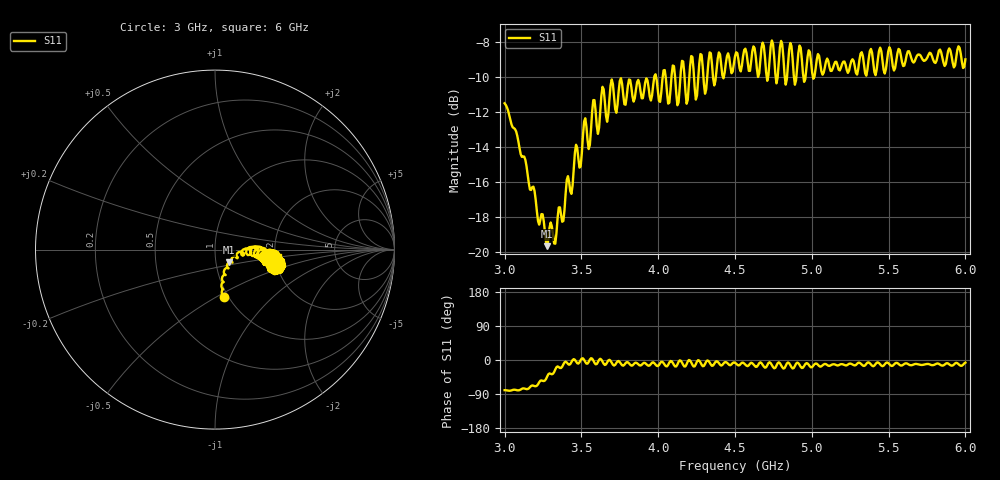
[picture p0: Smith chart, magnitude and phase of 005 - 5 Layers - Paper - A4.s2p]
!  02/07/2025  15:59:35
! Ref Plane: 0.000 mm
# MHZ S MA R  50
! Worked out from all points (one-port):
!   401 points, 3 GHz to 6 GHz, reference 50 ohm
!   lowest |S11| = -19.7 dB at 3.277 GHz (marker M1), VSWR 1.23, Z = 57.5 - j8.3 ohm
!   |S11| at or under -10 dB: start of sweep to 3.975 GHz; 3.986 GHz to 4.029 GHz (43.65 MHz wide, 1.09 % of centre); 4.048 GHz to 4.087 GHz (38.09 MHz wide, 0.936 % of centre)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
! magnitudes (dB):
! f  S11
! 3 GHz  -11.5
! 3.277 GHz  -19.7
! 3.375 GHz  -18.3
! 3.465 GHz  -13.9
! 3.547 GHz  -14.1
! 3.578 GHz  -11.3
! 3.607 GHz  -13.3
! 3.638 GHz  -10.6
! 3.667 GHz  -12.6
! 3.75 GHz  -10.2
! 4.013 GHz  -11.4
! 4.043 GHz  -9.6
! 4.065 GHz  -11.5
! 4.095 GHz  -9.4
! 4.125 GHz  -11.6
! 4.155 GHz  -9.1
! 4.185 GHz  -11.5
! 4.215 GHz  -8.8
! 4.245 GHz  -11.3
! 4.275 GHz  -8.7
! 4.305 GHz  -11.0
! 4.335 GHz  -8.6
! 4.365 GHz  -10.5
! 4.5 GHz  -8.8
! 4.875 GHz  -9.0
! 5.25 GHz  -9.3
! 5.625 GHz  -8.6
! 6 GHz  -9.0
